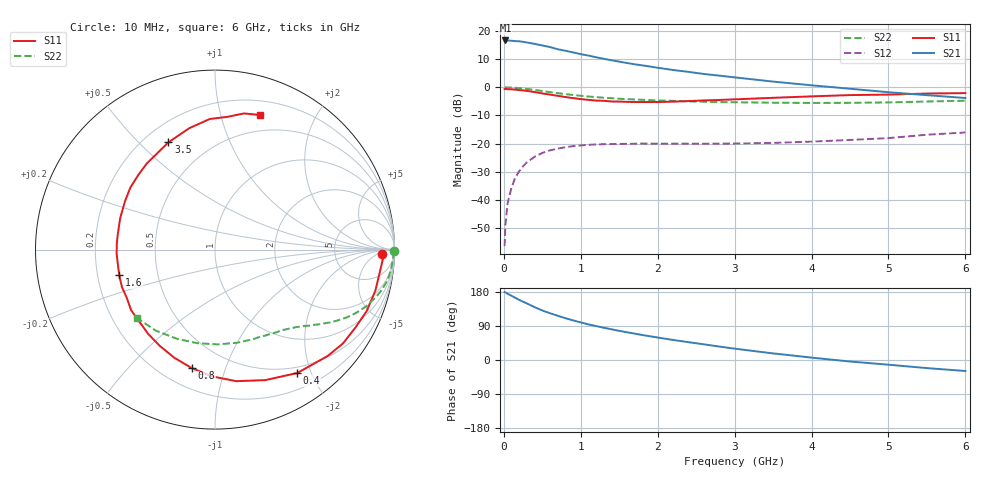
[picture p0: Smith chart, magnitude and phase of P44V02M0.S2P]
! SIEMENS Small Signal Semiconductors
! BFP182
! Si NPN RF Bipolar Junction Transistor in SOT143
! VCE = 4 V  IC = 2 mA
! Common Emitter S-Parameters:  March  1996
# GHz  S  MA  R  50
!  f  S11  S21  S12  S22
! GHz  MAG  ANG  MAG  ANG  MAG  ANG  MAG  ANG
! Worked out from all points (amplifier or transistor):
!   36 points, 10 MHz to 6 GHz, reference 50 ohm
!   highest |S21| = 16.7 dB at 20 MHz (marker M1)
!   |S21| within 3 dB of that: start of sweep to 684.9 MHz
!   unconditionally stable (mu >= 1): 2.208 GHz to end of sweep
!   at 250 MHz: K = 0.13, MSG = 22.1 dB, |S12| = -28.0 dB
!   at 1.4 GHz: K = 0.67, MSG = 14.9 dB, |S12| = -20.2 dB
!   at 6 GHz: K = 1.01, MAG = 5.6 dB, |S12| = -16.1 dB
!   lowest NFmin = 1.10 dB at 450 MHz
!   S11 on the Smith chart (normalised r, x): 10 MHz: 25, -9; 400 MHz: 0.41, -1.80; 800 MHz: 0.32, -0.77; 1.6 GHz: 0.29, -0.12; 3.5 GHz: 0.30, +0.61; 6 GHz: 0.33, +1.33
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0.01  0.9318 -1.4  6.791 179.2  0.0015 93.4  0.996 -0.6
0.02  0.937 -3.1  6.819 178.4  0.0036 82.0  0.9937 -1.2
0.05  0.9273 -7.5  6.783 174.7  0.0088 88.5  0.9936 -2.8
0.1  0.9222 -14.4  6.745 169.4  0.0166 80.1  0.988 -5.8
0.2  0.8943 -29.4  6.598 158.6  0.0324 72.3  0.9692 -11.3
0.25  0.8839 -36.3  6.444 153.6  0.0396 68.8  0.9538 -13.9
0.4  0.8264 -56.3  5.932 139.4  0.0583 58.3  0.9004 -20.5
0.5  0.7794 -68.9  5.559 130.7  0.0682 51.4  0.8603 -24.3
0.6  0.7427 -80.8  5.202 123.4  0.0757 46.2  0.8233 -27.4
0.7  0.707 -91.1  4.764 116.7  0.0813 41.7  0.7883 -30.1
0.8  0.6732 -101.0  4.476 110.3  0.0862 37.4  0.7579 -32.4
1  0.6183 -119.9  3.894 99.1  0.0926 30.7  0.7082 -36.1
1.1  0.5991 -128.5  3.668 93.9  0.0951 28.1  0.6868 -37.7
1.3  0.5764 -144.2  3.217 85.1  0.0975 23.5  0.6536 -40.6
1.6  0.5523 -165.0  2.71 73.2  0.0992 18.9  0.6181 -44.7
1.9  0.5479 176.6  2.344 62.6  0.0999 15.8  0.5923 -48.9
2.2  0.5568 161.5  2.033 52.9  0.0998 14.4  0.5751 -53.2
2.8  0.5969 135.4  1.615 35.4  0.0999 13.6  0.546 -63.1
3.5  0.6514 113.5  1.265 17.4  0.1029 14.6  0.5331 -76.9
4.5  0.7282 92.3  0.945 -4.0  0.1162 17.5  0.5306 -100.7
5.5  0.7756 78.0  0.726 -21.4  0.1438 17.9  0.5595 -126.3
6  0.7902 71.7  0.646 -29.0  0.1575 15.3  0.5786 -138.9
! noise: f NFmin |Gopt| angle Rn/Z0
0.45  1.1  0.42  29  0.36
0.9  1.2  0.4  58  0.3
1.8  1.85  0.32  126  0.22
